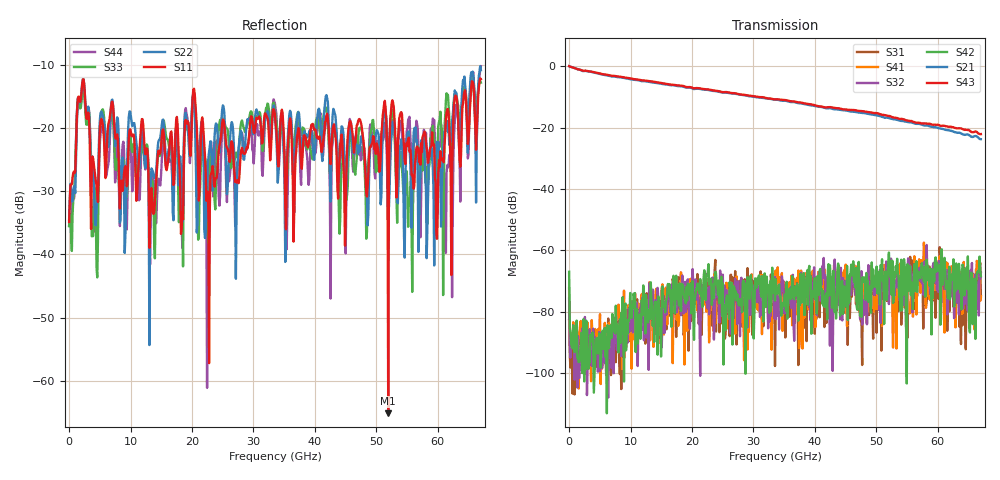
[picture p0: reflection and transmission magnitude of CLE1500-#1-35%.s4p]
!Keysight Technologies,N5247B,US50470101,A.16.20.02
!Date: Thursday, March 13, 2025 10:18:15
!Correction: S11(C  4-Port  )
!S12(C  4-Port  )
!S13(C  4-Port  )
!S14(C  4-Port  )
!S21(C  4-Port  )
!S22(C  4-Port  )
!S23(C  4-Port  )
!S24(C  4-Port  )
!S31(C  4-Port  )
!S32(C  4-Port  )
!S33(C  4-Port  )
!S34(C  4-Port  )
!S41(C  4-Port  )
!S42(C  4-Port  )
!S43(C  4-Port  )
!S44(C  4-Port  )
!S4P File: Measurements: <S11,S12,S13,S14>,
!<S21,S22,S23,S24>,
!<S31,S32,S33,S34>,
!<S41,S42,S43,S44>:
# Hz S  dB  R 50
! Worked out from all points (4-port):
!   601 points, 10 MHz to 67 GHz, reference 50 ohm
!   strongest paths, dB at 10 MHz, 16.76 GHz, 33.51 GHz, 50.25 GHz, 67 GHz:
!     S43: 0.0, -6.0, -10.8, -15.4, -22.1
!     S21: 0.0, -6.2, -10.9, -16.1, -23.8
!     S42: -67.0, -73.0, -76.4, -68.6, -68.5
!     S32: -75.7, -82.7, -68.7, -71.6, -67.4
!     S41: -82.9, -73.6, -69.2, -71.4, -75.0
!     S31: -72.3, -76.1, -97.8, -73.0, -75.2
!   lowest |S11| = -65.2 dB at 51.93 GHz (marker M1), VSWR 1.00, Z = 50 + j0.0485 ohm
!   |S11| at or under -10 dB: start of sweep to end of sweep
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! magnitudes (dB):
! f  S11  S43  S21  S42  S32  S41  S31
! 10 MHz  -34.9  0.0  0.0  -67.0  -75.7  -82.9  -72.3
! 2.243 GHz  -12.3  -1.5  -1.6  -95.8  -91.0  -98.4  -90.6
! 4.364 GHz  -28.5  -2.1  -2.2  -89.2  -90.2  -91.3  -98.1
! 5.369 GHz  -18.9  -2.6  -2.7  -87.4  -98.4  -98.6  -92.6
! 13.74 GHz  -33.6  -5.1  -5.3  -80.2  -81.8  -91.5  -76.6
! 51.93 GHz  -65.2  -16.2  -16.8  -64.0  -68.5  -65.5  -72.3
! 67 GHz  -12.3  -22.1  -23.8  -68.5  -67.4  -75.0  -75.2
